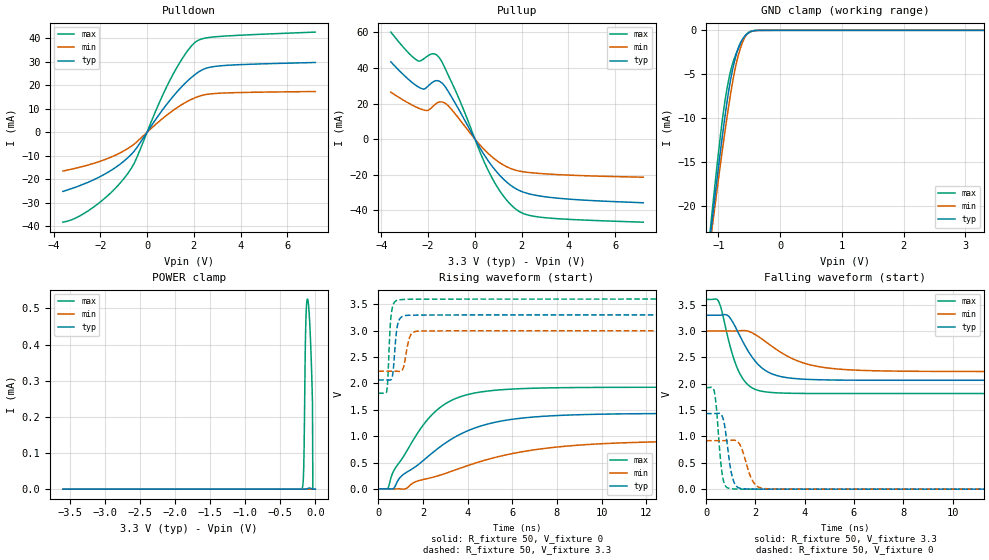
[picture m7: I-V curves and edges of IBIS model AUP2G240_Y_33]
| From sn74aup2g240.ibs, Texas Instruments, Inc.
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[Model]   AUP2G240_Y_33
Model_type  3-state
Enable   Active-Low
Vref =   0
Rref =   1E6
Cref =   30p
Vmeas =   1.65
| variable   typ   min   max
C_comp   2.02pF   1.81pF   2.42pF
| C_pullup   3.01pF   2.00pF   3.87pF
| C_pulldown   2.32pF   2.09pF   2.77pF
| C_tri-state   2.02pF   1.81pF   2.42pF
[Temperature Range]   40   100   -40
| Ambient temperature   25   85   -40
[Voltage range]   3.3   3   3.6
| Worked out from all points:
|   slope of the pulldown table from 0 to 0.495 V, typ, clamps not added: 68.4 ohm
|   slope of the pullup table from 0 to 0.495 V, typ, clamps not added: 45.8 ohm
|   GND clamp passes 1 mA (typ) near -0.61 V on its own axis
|   rising waveform, R_fixture 50, V_fixture 0: 20-80 % time 3.1ns typ, 4.78ns min, 2.01ns max; typ from 0 V to 1.43 V
|   falling waveform, R_fixture 50, V_fixture 3.3: 20-80 % time 1.02ns typ, 1.74ns min, 687ps max; typ from 3.3 V to 2.07 V
|   rising waveform, R_fixture 50, V_fixture 3.3: 20-80 % time 156ps typ, 208ps min, 125ps max; typ from 2.07 V to 3.3 V
|   falling waveform, R_fixture 50, V_fixture 0: 20-80 % time 264ps typ, 386ps min, 206ps max; typ from 1.43 V to 0 V
[GND Clamp]
| AUP2G240_Y_33
|   Voltage   I(typ)   I(min)   I(max)
-3.6V     -191.7mA   -177.9mA   -208.5mA
-1.125V   -23mA      -23.74mA   -22.15mA
-1.1V     -21.49mA   -22.35mA   -20.45mA
-1.075V   -19.98mA   -20.98mA   -18.78mA
-940mV    -12.21mA   -13.79mA   -10.35mA
-885mV    -9.313mA   -11.02mA   -7.613mA
-820mV    -6.304mA   -7.971mA   -5.14mA
-740mV    -3.515mA   -4.748mA   -3.135mA
-665mV    -1.768mA   -2.52mA    -1.842mA
-580mV    -733.4uA   -902.1uA   -734uA
-495mV    -220.6uA   -214.9uA   -155.7uA
3.3V      266.1pA    1.888nA    65.76pA
[POWER Clamp]
| AUP2G240_Y_33
|   Voltage   I(typ)   I(min)   I(max)
-3.6V     2.099nA    3.355nA    947.7pA
-195mV    1.242nA    2.95nA     734.1nA
-165mV    9.029nA    6.255nA    59.57uA
-155mV    24.86nA    9.366nA    182.7uA
-145mV    71.27nA    14.65nA    357.5uA
-135mV    201.7nA    22.66nA    463.4uA
-110mV    1.637uA    47.38nA    526.1uA
-80mV     3.299uA    48.09nA    461.7uA
-45mV     439nA      7.841nA    276.4uA
-40mV     578.7pA    4.7nA      236.1uA
-35mV     511pA      2.8nA      84.9pA
0V        0A         0A         0A
[Pulldown]
| AUP2G240_Y_33
|   Voltage   I(typ)   I(min)   I(max)
-3.6V     -25.17mA   -16.49mA   -38.29mA
-2.98V    -23.1mA    -15.14mA   -36.16mA
-2.195V   -19.8mA    -12.96mA   -31.18mA
-1.455V   -15.7mA    -10.21mA   -24.85mA
-850mV    -11.09mA   -7.079mA   -17.9mA
-485mV    -7.202mA   -4.495mA   -11.84mA
415mV     6.109mA    3.748mA    10.09mA
1.015V    14.06mA    8.579mA    22.82mA
1.6V      20.58mA    12.45mA    32.78mA
2.085V    24.83mA    14.83mA    38.52mA
3.09V     28.26mA    16.63mA    40.81mA
7.2V      29.73mA    17.36mA    42.67mA
[Pullup]
| AUP2G240_Y_33
|   Voltage   I(typ)   I(min)   I(max)
-3.6V     43.42mA    26.37mA    60.15mA
-2.72V    32.16mA    19.36mA    46.86mA
-2.285V   28.42mA    16.73mA    44.27mA
-2.015V   29.68mA    16.11mA    46.8mA
-1.81V    32mA       18.22mA    47.98mA
-1.495V   32.32mA    20.91mA    45.21mA
-1.11V    26.06mA    18.3mA     35.01mA
620mV     -13.19mA   -8.73mA    -19.02mA
1.19V     -22.14mA   -14.34mA   -31.52mA
1.765V    -27.99mA   -17.58mA   -39.54mA
2.955V    -32.36mA   -19.51mA   -44.15mA
7.2V      -35.8mA    -21.44mA   -46.72mA
[Ramp]
| AUP2G240_Y_33
| variable   typ   min   max
dV/dt_r   0.86/3.10E-09   0.55/4.80E-09   1.16/2.02E-09
dV/dt_f   0.75/1.02E-09   0.47/1.75E-09   1.08/6.90E-10
R_load = 50
[Rising Waveform]
| AUP2G240_Y_33
R_fixture =   50
C_fixture =   0
L_fixture =   0
V_fixture =   0
V_fixture_min = 0
V_fixture_max = 0
|   Time   V(typ)   V(min)   V(max)
0s        12.11nV    31.97nV    1.283nV
433ps     330.1uV    -16.95uV   11.58mV
733ps     31.13mV    267.4uV    372.2mV
1.057ns   249.8mV    -2.53mV    567.4mV
2.345ns   655.1mV    209.9mV    1.379V
3.085ns   892.1mV    305.3mV    1.634V
3.977ns   1.097V     438.2mV    1.786V
5.977ns   1.319V     668.4mV    1.893V
8.869ns   1.405V     826.7mV    1.922V
18.41ns   1.434V     916.2mV    1.928V
[Falling Waveform]
| AUP2G240_Y_33
R_fixture =   50
C_fixture =   0
L_fixture =   0
V_fixture =   3.3
V_fixture_min = 3
V_fixture_max = 3.6
|   Time   V(typ)   V(min)   V(max)
0s        3.3V       3V         3.6V
493ps     3.299V     3V         3.572V
629ps     3.303V     3V         3.394V
909ps     3.282V     3V         2.829V
1.181ns   3.085V     3V         2.398V
1.477ns   2.811V     3.009V     2.105V
2.269ns   2.299V     2.847V     1.857V
3.713ns   2.094V     2.434V     1.817V
5.381ns   2.07V      2.278V     1.814V
18.41ns   2.066V     2.232V     1.814V
[Rising Waveform]
| AUP2G240_Y_33
R_fixture =   50
C_fixture =   0
L_fixture =   0
V_fixture =   3.3
V_fixture_min = 3
V_fixture_max = 3.6
|   Time   V(typ)   V(min)   V(max)
0s        2.066V     2.232V     1.814V
373ps     2.066V     2.232V     1.833V
425ps     2.066V     2.232V     2.033V
521ps     2.064V     2.232V     2.965V
589ps     2.077V     2.232V     3.328V
897ps     3.162V     2.229V     3.583V
1.125ns   3.278V     2.3V       3.593V
1.437ns   3.294V     2.906V     3.596V
1.741ns   3.296V     2.99V      3.597V
18.41ns   3.3V       3V         3.6V
[Falling Waveform]
| AUP2G240_Y_33
R_fixture =   50
C_fixture =   0
L_fixture =   0
V_fixture =   0
V_fixture_min = 0
V_fixture_max = 0
|   Time   V(typ)   V(min)   V(max)
0s        1.434V     920.1mV    1.928V
325ps     1.435V     920mV      1.875V
417ps     1.437V     919.9mV    1.551V
657ps     1.379V     919.8mV    274.4mV
921ps     613.9mV    923.5mV    16.18mV
1.081ns   201.3mV    928.9mV    5.908mV
1.261ns   42.55mV    908.7mV    2.211mV
1.885ns   1.767mV    159.5mV    391.6uV
2.333ns   749.5uV    12.4mV     173.2uV
18.41ns   27.55nV    91.37nV    13.73nV
